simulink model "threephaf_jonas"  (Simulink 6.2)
settings: Solver=ode23  StartTime=0  StopTime=0.05  FixedStep=0.000001  MaxStep=2e-5  RelTol=1e-3
undefined symbols (not defined in the file or in its folder): Cdc, di, DiscIntNeverNeededParam, Element, L, R, Symmetrized, Tf, Ts, Udc, Upp, Warning, Yes
libraries: simulink x12
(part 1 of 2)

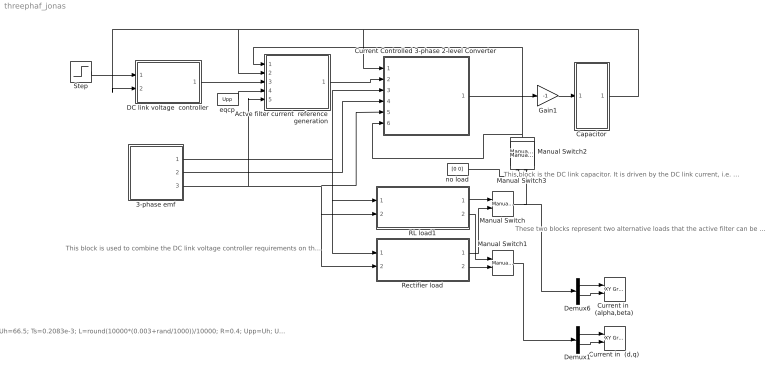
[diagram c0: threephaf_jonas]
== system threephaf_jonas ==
  note: These two blocks represent two alternative loads that the active filter can be used with.
  note: This block is the DC link capacitor. It is driven by the DC link current, i.e. the DC link voltage is the integral of the DC link current divided by the capacitance.
  note: This block is used to combine the DC link voltage controller requirements on the filter current with the components of the load current that can be filtered out.
  note: Uh=66.5; Ts=0.2083e-3; L=round(10000*(0.003+rand/1000))/10000; R=0.4; Upp=Uh; Udc=250; Cdc=0.0011; di=3; Tf=1/(2*pi*30);
  3-phase emf : Subsystem  mask{Upp=Upp, freq=50, Tc=0.1e-3}
      mask prompts: Upp "U_phase_to_phase [RMS]"; freq "Frequency"; Tc "Sampling time"
  Actve filter current  reference generation : Subsystem
  Capacitor : Subsystem
  Current Controlled 3-phase 2-level Converter : Subsystem
  Current in  (alpha,beta) : simulink/Sinks/XY Graph  xmin=-20  xmax=20  ymin=-20  ymax=20  st=-1
  Current in  (d,q) : simulink/Sinks/XY Graph  xmin=-20  xmax=20  ymin=-20  ymax=20  st=-1
  DC link voltage  controller : Subsystem  mask{Kp=Cdc/3/Tf, Ti=9*Tf, Ttc=Ts, Limitoutput=Yes, Out_max=20, Out_min=-20}
      mask prompts: Kp "Gain"; Ti "Integral time constant"; Ttc "Controller Sampling Time"; Limitoutput "Limit the output"; Out_max "Max Controller Output (if limited)     INCLUDES Anti Windup !!"; Out_min "Min Controller Output (if limited)     INCLUDES Anti Windup !!"
  Demux1 : Demux  Outputs=2
  Demux6 : Demux  Outputs=2
  Gain1 : Gain  Gain=-1
  Manual Switch : simulink/Signal Routing/Manual Switch  sw=1  action=0
  Manual Switch1 : simulink/Signal Routing/Manual Switch  sw=1  action=0
  Manual Switch2 : simulink/Signal Routing/Manual Switch  Orientation=up  sw=1  action=0
  Manual Switch3 : simulink/Signal Routing/Manual Switch  Orientation=up  sw=0  action=0
  RL load1 : Subsystem  mask{Ra=5, Rb=5, Rc=5, La=0.005, Lb=0.005, Lc=0.005, Imax=1}
      mask prompts: Ra "Ra [Ohm]"; Rb "Rb [Ohm]"; Rc "Rc [Ohm]"; La "La [H]"; Lb "Lb [H]"; Lc "Lc [H]"; Imax "Current when saturation starts"
  Rectifier load : Subsystem
  Step : Step  Time=0.005  Before=250  After=260  SampleTime=0
  eqcp : Constant  Value=Upp
  no load : Constant  Value=[0 0]
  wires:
  Gain1/1 -> Capacitor/1(iC)
  Current Controlled 3-phase 2-level Converter/1(idc) -> Gain1/1
  DC link voltage  controller/1(Out) -> Actve filter current  reference generation/3(idc*)
  eqcp/1 -> Actve filter current  reference generation/4(eqcp)
  Step/1 -> DC link voltage  controller/1(Ref)
  Capacitor/1(Udc) -> Actve filter current  reference generation/2(Udc), DC link voltage  controller/2(Act), Current Controlled 3-phase 2-level Converter/1(Udc)
  RL load1/1(i_load_ab) -> Manual Switch/1
  Rectifier load/1(i_load_ab) -> Manual Switch/2
  Rectifier load/2(i_load_dq) -> Manual Switch1/2
  RL load1/2(i_load_dq) -> Manual Switch1/1
  Actve filter current  reference generation/1(idq*) -> Current Controlled 3-phase 2-level Converter/2(idq*)
  3-phase emf/1(e_line) -> Current Controlled 3-phase 2-level Converter/3(e_line), Rectifier load/1(u_line), RL load1/1(u_line)
  3-phase emf/2(Psi_line) -> Current Controlled 3-phase 2-level Converter/4(Psi_line)
  3-phase emf/3(Theta_line) -> Actve filter current  reference generation/5(Theta), Current Controlled 3-phase 2-level Converter/5(Theta_line), Rectifier load/2(Theta), RL load1/2(Theta)
  Manual Switch/1 -> Manual Switch2/2, Demux6/1
  no load/1 -> Manual Switch2/1
  Manual Switch2/1 -> Actve filter current  reference generation/1(i_load), Current Controlled 3-phase 2-level Converter/6(Load current in a/b)
  Manual Switch1/1 -> Demux1/1
  Demux6/1 -> Current in  (alpha,beta)/1
  Demux6/2 -> Current in  (alpha,beta)/2
  Demux1/1 -> Current in  (d,q)/1
  Demux1/2 -> Current in  (d,q)/2

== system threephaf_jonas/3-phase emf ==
  note: Power invariant emf vector on alpha/beta frame
  Cos Fcn : Fcn  Expr=cos(2*pi*(u(2))*u(1))
  Digital Clock : DigitalClock  SampleTime=Tc
  Mux : Mux  Inputs=2
  Mux1 : Mux  Inputs=2
  Product : Product
  Sine Fcn : Fcn  Expr=sin(2*pi*(u(2))*u(1)-pi)
  frequency : Constant  Value=freq
  integrator : Subsystem
  line voltage : Constant  Value=Upp
  rec_to_pol : Subsystem
  e_line : Outport  InitialOutput=0
  Psi_line : Outport  Port=2  InitialOutput=0
  Theta_line : Outport  Port=3  InitialOutput=0
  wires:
  Product/1 -> e_line/1, integrator/1(In1)
  Mux1/1 -> Product/1
  Cos Fcn/1 -> Mux1/2
  Sine Fcn/1 -> Mux1/1
  Mux/1 -> Cos Fcn/1, Sine Fcn/1
  Digital Clock/1 -> Mux/1
  frequency/1 -> Mux/2
  line voltage/1 -> Product/2
  integrator/1(Out1) -> Psi_line/1, rec_to_pol/1(rect)
  rec_to_pol/2(angle) -> Theta_line/1

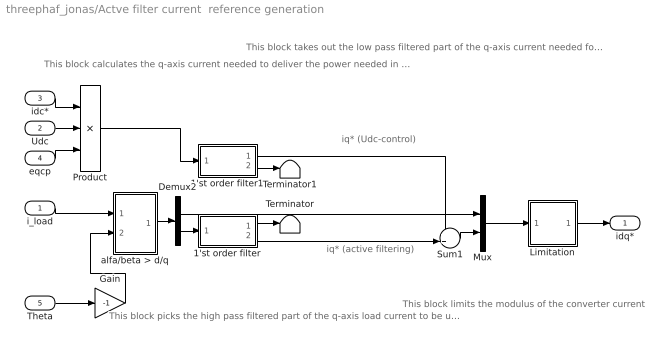
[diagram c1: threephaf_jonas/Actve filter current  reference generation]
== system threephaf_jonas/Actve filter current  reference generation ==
  note: iq* (Udc-control)
  note: iq* (active filtering)
  note: This block calculates the q-axis current needed to deliver the power needed in the dc-link for correcting the DC link voltage error, as ordered by the DC link voltage controller
  note: This block takes out the low pass filtered part of the q-axis current needed for DC link voltage control
  note: This block picks the high pass filtered part of the q-axis load current to be used as reference for the q-axis together with the low pass filtered part of the DC link voltage controller output.
  note: This block limits the modulus of the converter current
  i_load : Inport  Port=1  LatchInput=off
  Udc : Inport  Port=2  LatchInput=off
  idc* : Inport  Port=3  LatchInput=off
  eqcp : Inport  Port=4  LatchInput=off
  Theta : Inport  Port=5  LatchInput=off
  1'st order filter : Subsystem
  1'st order filter1 : Subsystem
  Demux2 : Demux  Outputs=2
  Gain : Gain  Gain=-1
  Limitation : Subsystem
  Mux : Mux  Inputs=2
  Product : Product  Inputs=**/
  Sum1 : Sum  Inputs=++|
  Terminator : Terminator
  Terminator1 : Terminator
  alfa/beta > d/q : Subsystem
  idq* : Outport
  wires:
  i_load/1 -> alfa/beta > d/q/1(vect)
  Gain/1 -> alfa/beta > d/q/2(angle)
  Theta/1 -> Gain/1
  Demux2/1 -> Mux/1
  Demux2/2 -> 1'st order filter/1(In)
  1'st order filter/1(OutLP) -> Terminator/1
  alfa/beta > d/q/1(Out) -> Demux2/1
  1'st order filter/2(OutHP) -> Sum1/2
  Sum1/1 -> Mux/2
  Limitation/1(i*lim) -> idq*/1
  1'st order filter1/1(OutLP) -> Sum1/1
  eqcp/1 -> Product/3
  Udc/1 -> Product/2
  Product/1 -> 1'st order filter1/1(In)
  idc*/1 -> Product/1
  1'st order filter1/2(OutHP) -> Terminator1/1
  Mux/1 -> Limitation/1(i*)

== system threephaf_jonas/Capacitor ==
  iC : Inport  Port=1  LatchInput=off
  Gain : Gain  Gain=1/Cdc
  Integrator : Integrator  InitialCondition=Udc
  Udc : Outport
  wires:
  Gain/1 -> Integrator/1
  iC/1 -> Gain/1
  Integrator/1 -> Udc/1

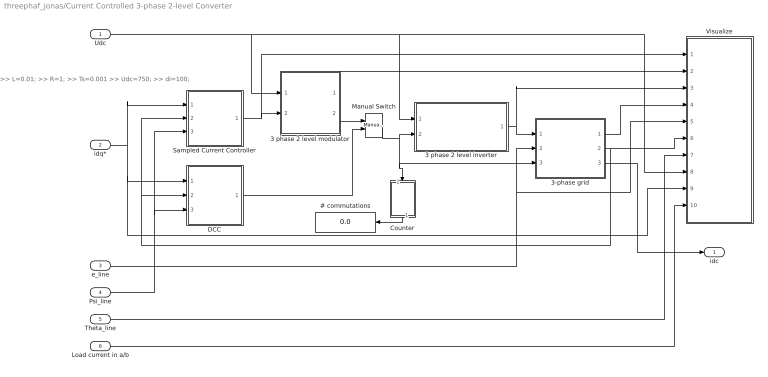
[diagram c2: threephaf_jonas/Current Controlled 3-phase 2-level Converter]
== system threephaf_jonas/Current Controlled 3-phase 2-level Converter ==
  note: >> L=0.01; >> R=1; >> Ts=0.001 >> Udc=750; >> di=100;
  Udc : Inport  Port=1  LatchInput=off
  idq* : Inport  Port=2  LatchInput=off
  e_line : Inport  Port=3  LatchInput=off
  Psi_line : Inport  Port=4  LatchInput=off
  Theta_line : Inport  Port=5  LatchInput=off
  Load current in a/b : Inport  Port=6  LatchInput=off
  # commutations : Display
  3 phase 2 level inverter : Subsystem
  3 phase 2 level modulator : Subsystem  mask{type=Symmetrized, Random=Fixed frequency, Ts=Ts}
      mask prompts: type "Sinus, Symmetrized or Minimum switch modulation"; Random "Fixed or random modulation?"; Ts "Sampling interval"
      mask help: Carrier Wave modulator that uses either fixed frequency modulation or random modulation. The fixed frequency modulation uses 1/(2Ts) as modulation frequency. The random modulation selects the modulatio frequency by random every sampling instant. The selection uses either 1/Ts, 1/(2Ts) or 1/(3Ts) as carrier wave frequency.
  3-phase grid : Subsystem  mask{L=L, R=R}
      mask prompts: L "Inductance [H]"; R "Resistance [ohm]"
  Counter : Subsystem  Orientation=down
  DCC : Subsystem
  Manual Switch : simulink/Signal Routing/Manual Switch  sw=1  action=0
  Sampled Current Controller : Subsystem  mask{R=R, L=L, Kp=(L/Ts+R/2), Ti=L/R+Ts/2, Ts=Ts, Umax=Udc, Umin=-Udc, SlowFast=Fast computer}
      mask prompts: R "Load resistance"; L "Load inductance"; Kp "Controller gain"; Ti "Integral Time Constant"; Ts "Sampling time [s]"; Umax "Max output signal"; Umin "Min output signal"; SlowFast "Controller type"
  Visualize : Subsystem
  idc : Outport
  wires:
  3 phase 2 level inverter/1(va,b,c) -> 3-phase grid/1(va,b,c), Visualize/3(v)
  Sampled Current Controller/1(u*) -> 3 phase 2 level modulator/2(uabc*), Visualize/1(u*)
  Udc/1 -> 3 phase 2 level modulator/1(Udc), 3 phase 2 level inverter/1(Udc), Visualize/8(Udc)
  Counter/1(#) -> # commutations/1
  3 phase 2 level modulator/2(sa,b,c) -> Manual Switch/1
  Manual Switch/1 -> 3 phase 2 level inverter/2(sa,b,c), Counter/1(sa,b,c), 3-phase grid/3(s)
  DCC/1(sa,b,c) -> Manual Switch/2
  3 phase 2 level modulator/1(mod) -> Visualize/2(mod)
  e_line/1 -> 3-phase grid/2(e_line), Visualize/5(e)
  3-phase grid/1(u_ab) -> Visualize/4("u ")
  3-phase grid/2(i_ab) -> Visualize/6(i), DCC/2(Act_ab), Sampled Current Controller/2(Act_ab)
  Theta_line/1 -> Visualize/7(theta)
  Psi_line/1 -> DCC/3(psi), Sampled Current Controller/3(psi)
  idq*/1 -> Sampled Current Controller/1(Ref_dq), DCC/1(Ref_dq), Visualize/9(i*dq)
  3-phase grid/3(i_dc) -> idc/1
  Load current in a/b/1 -> Visualize/10(Load current in a/b)

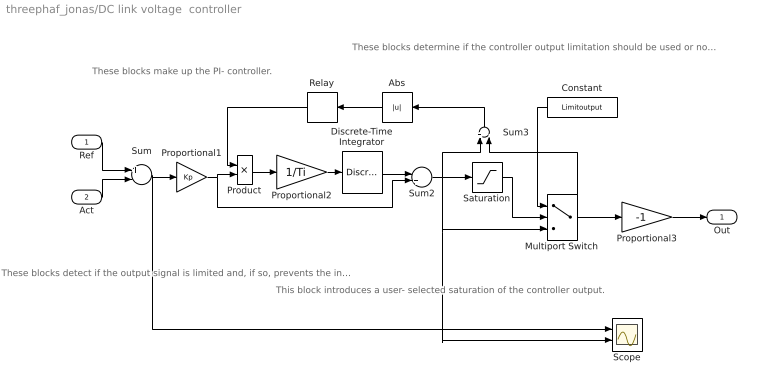
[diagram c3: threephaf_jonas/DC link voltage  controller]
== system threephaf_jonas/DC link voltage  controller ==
  note: These blocks make up the PI- controller.
  note: These blocks detect if the output signal is limited and, if so, prevents the integrator from integrating.
  note: This block introduces a user- selected saturation of the controller output.
  note: These blocks determine if the controller output limitation should be used or not.
  Ref : Inport  Port=1  LatchInput=off
  Act : Inport  Port=2  LatchInput=off
  Abs : Abs  Orientation=left
  Constant : Constant  Orientation=left  Value=Limitoutput
  Discrete-Time Integrator : DiscreteIntegrator  SampleTime=Ttc  ICPrevOutput=DiscIntNeverNeededParam  ICPrevScaledInput=DiscIntNeverNeededParam
  Multiport Switch : MultiPortSwitch  Inputs=2
  Product : Product
  Proportional1 : Gain  Gain=Kp
  Proportional2 : Gain  Gain=1/Ti
  Proportional3 : Gain  Gain=-1
  Relay : Relay  Orientation=left  OnOutputValue=0  OffOutputValue=1
  Saturation : Saturate  UpperLimit=Out_max  LowerLimit=Out_min
  Scope : Scope  NumInputPorts=2
  Sum : Sum  Inputs=+-
  Sum2 : Sum
  Sum3 : Sum  Orientation=up  Inputs=+-
  Out : Outport
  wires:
  Sum/1 -> Proportional1/1, Scope/1
  Discrete-Time Integrator/1 -> Sum2/1
  Proportional1/1 -> Product/2, Sum2/2
  Proportional2/1 -> Discrete-Time Integrator/1
  Sum2/1 -> Saturation/1, Sum3/1, Multiport Switch/3, Scope/2
  Product/1 -> Proportional2/1
  Sum3/1 -> Abs/1
  Abs/1 -> Relay/1
  Relay/1 -> Product/1
  Ref/1 -> Sum/1
  Act/1 -> Sum/2
  Saturation/1 -> Multiport Switch/2
  Constant/1 -> Multiport Switch/1
  Multiport Switch/1 -> Sum3/2, Proportional3/1
  Proportional3/1 -> Out/1

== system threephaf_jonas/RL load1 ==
  u_line : Inport  Port=1  LatchInput=off
  Theta : Inport  Port=2  LatchInput=off
  Gain1 : Gain  Gain=-1
  Load : Subsystem  mask{La=La, Lb=Lb, Lc=Lc, Imax=Imax, Ra=Ra, Rb=Rb, Rc=Rc}
      mask prompts: Imax "Inductor current for saturation"
  "a/b -> d/q1" : Subsystem
  abc Ü> vector : Subsystem
  vector to abc2 : Subsystem
  i_load_ab : Outport
  i_load_dq : Outport  Port=2
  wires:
  vector to abc2/1(a) -> Load/1(a)
  vector to abc2/2(b) -> Load/2(b)
  vector to abc2/3(c) -> Load/3(c)
  Load/1(ia) -> abc Ü> vector/1(a)
  Load/2(ib) -> abc Ü> vector/2(b)
  Load/3(ic) -> abc Ü> vector/3(c)
  u_line/1 -> vector to abc2/1(vect)
  abc Ü> vector/1(vect) -> i_load_ab/1, "a/b -> d/q1"/1(vect)
  Gain1/1 -> "a/b -> d/q1"/2(angle)
  Theta/1 -> Gain1/1
  "a/b -> d/q1"/1(Out) -> i_load_dq/1

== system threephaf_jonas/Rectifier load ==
  u_line : Inport  Port=1  LatchInput=off
  Theta : Inport  Port=2  LatchInput=off
  Gain1 : Gain  Gain=-1
  Load : Subsystem
  "a/b -> d/q1" : Subsystem
  abc Ü> vector : Subsystem
  vector to abc2 : Subsystem
  i_load_ab : Outport
  i_load_dq : Outport  Port=2
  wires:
  "a/b -> d/q1"/1(Out) -> i_load_dq/1
  Theta/1 -> Gain1/1
  Gain1/1 -> "a/b -> d/q1"/2(angle)
  vector to abc2/1(a) -> Load/1(a)
  vector to abc2/2(b) -> Load/2(b)
  vector to abc2/3(c) -> Load/3(c)
  Load/1(ia) -> abc Ü> vector/1(a)
  Load/2(ib) -> abc Ü> vector/2(b)
  Load/3(ic) -> abc Ü> vector/3(c)
  u_line/1 -> vector to abc2/1(vect)
  abc Ü> vector/1(vect) -> "a/b -> d/q1"/1(vect), i_load_ab/1

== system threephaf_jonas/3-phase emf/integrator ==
  note: Power invariant emf vector on alpha/beta frame
  In1 : Inport  Port=1  LatchInput=off
  Demux : Demux  Outputs=2
  Integrator1 : Integrator  InitialCondition=Upp/(2*pi*freq)
  Integrator2 : Integrator
  Mux : Mux  Inputs=2
  Out1 : Outport
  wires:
  In1/1 -> Demux/1
  Mux/1 -> Out1/1
  Integrator2/1 -> Mux/2
  Integrator1/1 -> Mux/1
  Demux/2 -> Integrator2/1
  Demux/1 -> Integrator1/1

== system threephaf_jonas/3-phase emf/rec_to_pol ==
  rect : Inport  Port=1  LatchInput=off
  Derivative : Derivative
  Gain : Gain  Gain=-1
  alfa/beta Ü> d/q : Subsystem
  "angle " : Fcn  Expr=atan2(u[2],u[1])
  "mod " : Fcn  Expr=sqrt(u[1]^2+u[2]^2)
  e : Outport  InitialOutput=0
  angle : Outport  Port=2  InitialOutput=0
  mod : Outport  Port=3  InitialOutput=0
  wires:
  "angle "/1 -> angle/1, Gain/1
  rect/1 -> "angle "/1, "mod "/1, Derivative/1
  "mod "/1 -> mod/1
  Gain/1 -> alfa/beta Ü> d/q/2(angle)
  Derivative/1 -> alfa/beta Ü> d/q/1(vect)
  alfa/beta Ü> d/q/1(Out) -> e/1

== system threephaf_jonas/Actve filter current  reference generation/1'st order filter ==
  In : Inport  Port=1  LatchInput=off
  Gain4 : Gain  Gain=1/Tf
  Integrator : Integrator
  Sum : Sum  Inputs=-+
  Sum4 : Sum  Inputs=+-
  OutLP : Outport
  OutHP : Outport  Port=2
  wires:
  Sum4/1 -> Gain4/1
  Gain4/1 -> Integrator/1
  Integrator/1 -> OutLP/1, Sum4/2, Sum/1
  In/1 -> Sum4/1, Sum/2
  Sum/1 -> OutHP/1

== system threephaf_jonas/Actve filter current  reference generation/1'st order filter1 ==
  In : Inport  Port=1  LatchInput=off
  Gain : Gain  Gain=1/(Tf)
  Integrator : Integrator
  Sum : Sum  Inputs=-+
  Sum1 : Sum  Inputs=|+-
  OutLP : Outport
  OutHP : Outport  Port=2
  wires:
  Sum1/1 -> Gain/1
  Gain/1 -> Integrator/1
  Integrator/1 -> OutLP/1, Sum1/2, Sum/1
  In/1 -> Sum1/1, Sum/2
  Sum/1 -> OutHP/1

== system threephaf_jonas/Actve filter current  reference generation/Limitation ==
  note: abs(i*)
  note: Current Limiter
  i* : Inport  Port=1  LatchInput=off
  Constant : Constant  Value=20*sqrt(3/2)
  Fcn1 : Fcn  Expr=sqrt(u(1)^2+u(2)^2)
  Product : Product
  Product1 : Product
  Saturation : Saturate  UpperLimit=1  LowerLimit=0
  Sign4 : Signum
  Sum2 : Sum  Inputs=-+
  Switch4 : Switch
  i*lim : Outport
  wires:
  Saturation/1 -> Product1/2
  Product/1 -> Saturation/1
  Switch4/1 -> Product/1
  Fcn1/1 -> Product/2, Switch4/3, Sum2/2
  Sum2/1 -> Sign4/1
  Sign4/1 -> Switch4/2
  Constant/1 -> Switch4/1, Sum2/1
  i*/1 -> Product1/1, Fcn1/1
  Product1/1 -> i*lim/1

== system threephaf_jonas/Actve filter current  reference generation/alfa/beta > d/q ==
  vect : Inport  Port=1  LatchInput=off
  angle : Inport  Port=2  LatchInput=off
  Fcn : Fcn  Expr=u[1]*cos(u[3])-u[2]*sin(u[3])
  Fcn1 : Fcn  Expr=u[1]*sin(u[3])+u[2]*cos(u[3])
  Mux : Mux  Inputs=2
  Mux1 : Mux  Inputs=2
  Out : Outport  InitialOutput=0
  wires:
  vect/1 -> Mux/1
  angle/1 -> Mux/2
  Mux/1 -> Fcn/1, Fcn1/1
  Fcn/1 -> Mux1/1
  Fcn1/1 -> Mux1/2
  Mux1/1 -> Out/1

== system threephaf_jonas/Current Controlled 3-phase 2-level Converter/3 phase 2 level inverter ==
  Udc : Inport  Port=1  LatchInput=off
  sa,b,c : Inport  Port=2  LatchInput=off
  Demux : Demux  Outputs=3
  Gain : Gain  Gain=1/2
  Gain1 : Gain  Gain=-1/2
  Mux : Mux  Orientation=down  Inputs=3
  Switch : Switch
  Switch1 : Switch
  Switch2 : Switch
  va,b,c : Outport  Orientation=down  InitialOutput=0
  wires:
  Gain/1 -> Switch/1, Switch1/1, Switch2/1
  Gain1/1 -> Switch/3, Switch1/3, Switch2/3
  Udc/1 -> Gain1/1, Gain/1
  sa,b,c/1 -> Demux/1
  Demux/1 -> Switch/2
  Demux/2 -> Switch1/2
  Demux/3 -> Switch2/2
  Switch/1 -> Mux/1
  Switch1/1 -> Mux/2
  Switch2/1 -> Mux/3
  Mux/1 -> va,b,c/1

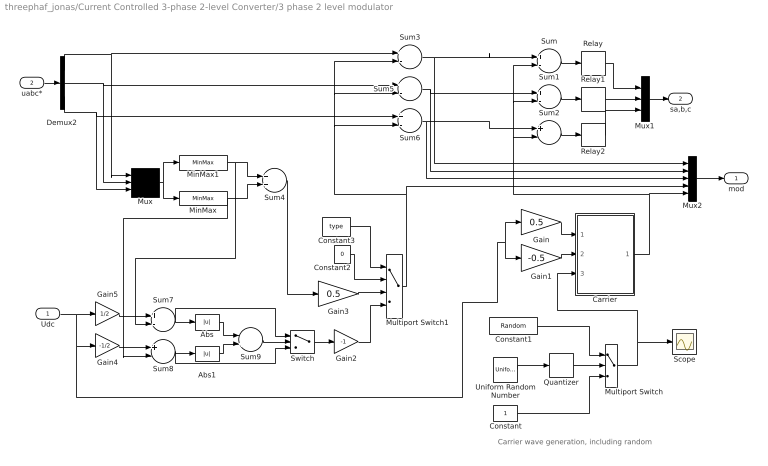
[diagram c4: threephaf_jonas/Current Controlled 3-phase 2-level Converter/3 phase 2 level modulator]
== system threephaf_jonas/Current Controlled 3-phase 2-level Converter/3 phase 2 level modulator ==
  note: Carrier wave generation, including random
  Udc : Inport  Port=1  LatchInput=off
  uabc* : Inport  Port=2  LatchInput=off
  Abs : Abs
  Abs1 : Abs
  Carrier : Subsystem
  Constant : Constant
  Constant1 : Constant  Value=Random
  Constant2 : Constant  Value=0
  Constant3 : Constant  Value=type
  Demux2 : Demux  Outputs=3
  Gain : Gain  Gain=0.5
  Gain1 : Gain  Gain=-0.5
  Gain2 : Gain  Gain=-1
  Gain3 : Gain  Gain=0.5
  Gain4 : Gain  Gain=-1/2
  Gain5 : Gain  Gain=1/2
  MinMax : MinMax
  MinMax1 : MinMax  Function=max
  Multiport Switch : MultiPortSwitch  Inputs=2
  Multiport Switch1 : MultiPortSwitch  Inputs=3
  Mux : Mux  Inputs=3
  Mux1 : Mux  Inputs=3
  Mux2 : Mux  Inputs=5
  Quantizer : Quantizer  QuantizationInterval=1
  Relay : Relay  OffOutputValue=-1
  Relay1 : Relay  OffOutputValue=-1
  Relay2 : Relay  OffOutputValue=-1
  Scope : Scope
  Sum{,1..3,5..8} (8 alike) : Sum  Inputs=+-
  Sum4 : Sum
  Sum9 : Sum  Inputs=-+
  Switch : Switch
  Uniform Random Number : UniformRandomNumber  Minimum=1  Maximum=3  Seed=0.9874  SampleTime=Ts
  mod : Outport  InitialOutput=0
  sa,b,c : Outport  Port=2  InitialOutput=0
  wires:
  Carrier/1(um) -> Sum2/2, Sum1/2, Sum/2, Mux2/5
  Gain1/1 -> Carrier/2(Umin)
  Gain/1 -> Carrier/1(Umax)
  Sum/1 -> Relay/1
  Relay1/1 -> Mux1/2
  Sum1/1 -> Relay1/1
  Relay2/1 -> Mux1/3
  Sum2/1 -> Relay2/1
  Sum3/1 -> Mux2/1, Sum/1
  Sum5/1 -> Mux2/2, Sum1/1
  Sum6/1 -> Mux2/3, Sum2/1
  Demux2/1 -> Sum3/1, Mux/1
  Demux2/2 -> Sum5/1, Mux/2
  Demux2/3 -> Sum6/1, Mux/3
  Mux/1 -> MinMax1/1, MinMax/1
  MinMax1/1 -> Sum4/1, Sum7/2
  MinMax/1 -> Sum4/2, Sum8/2
  Udc/1 -> Gain5/1, Gain4/1, Gain1/1, Gain/1
  Gain4/1 -> Sum8/1
  Sum7/1 -> Abs/1, Switch/1
  Sum8/1 -> Abs1/1, Switch/3
  Abs/1 -> Sum9/1
  Abs1/1 -> Sum9/2
  Sum9/1 -> Switch/2
  Sum4/1 -> Gain3/1
  Switch/1 -> Gain2/1
  Constant3/1 -> Multiport Switch1/1
  Constant2/1 -> Multiport Switch1/2
  Gain3/1 -> Multiport Switch1/3
  Gain2/1 -> Multiport Switch1/4
  Multiport Switch1/1 -> Sum5/2, Sum3/2, Sum6/2, Mux2/4
  Gain5/1 -> Sum7/1
  uabc*/1 -> Demux2/1
  Relay/1 -> Mux1/1
  Mux1/1 -> sa,b,c/1
  Mux2/1 -> mod/1
  Quantizer/1 -> Multiport Switch/2
  Uniform Random Number/1 -> Quantizer/1
  Constant/1 -> Multiport Switch/3
  Multiport Switch/1 -> Scope/1, Carrier/3(x)
  Constant1/1 -> Multiport Switch/1

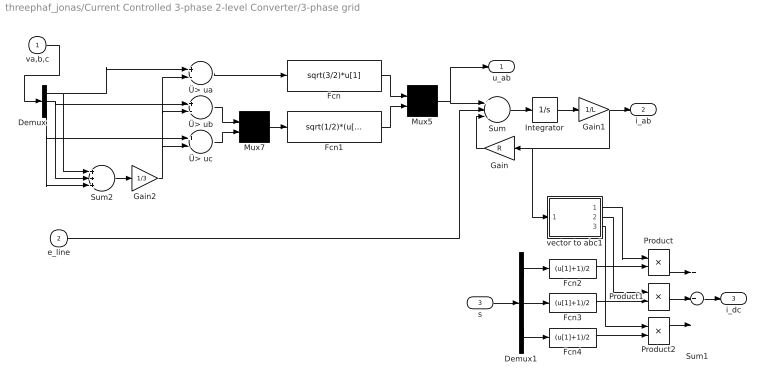
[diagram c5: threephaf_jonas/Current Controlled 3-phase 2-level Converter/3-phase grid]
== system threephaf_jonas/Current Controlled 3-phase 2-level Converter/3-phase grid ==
  va,b,c : Inport  Port=1  LatchInput=off
  e_line : Inport  Port=2  LatchInput=off
  s : Inport  Port=3  LatchInput=off
  Demux : Demux  Outputs=3
  Demux1 : Demux  Outputs=3
  Fcn : Fcn  Expr=sqrt(3/2)*u[1]
  Fcn1 : Fcn  Expr=sqrt(1/2)*(u[1]-u[2])
  Fcn2 : Fcn  Expr=(u[1]+1)/2
  Fcn3 : Fcn  Expr=(u[1]+1)/2
  Fcn4 : Fcn  Expr=(u[1]+1)/2
  Gain : Gain  Orientation=left  Gain=R
  Gain1 : Gain  Gain=1/L
  Gain2 : Gain  Gain=1/3
  Integrator : Integrator
  Mux5 : Mux  Inputs=2
  Mux7 : Mux  Inputs=2
  Product : Product
  Product1 : Product
  Product2 : Product
  Sum : Sum  Inputs=+--
  Sum1 : Sum  Inputs=+++
  Sum2 : Sum  Inputs=+++
  vector to abc1 : Subsystem
  Ü> ua : Sum  Inputs=+-
  Ü> ub : Sum  Inputs=+-
  Ü> uc : Sum  Inputs=+-
  u_ab : Outport  InitialOutput=0
  i_ab : Outport  Port=2  InitialOutput=0
  i_dc : Outport  Port=3
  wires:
  Gain1/1 -> i_ab/1, Gain/1, vector to abc1/1(vect)
  Integrator/1 -> Gain1/1
  Gain/1 -> Sum/3
  Sum/1 -> Integrator/1
  Fcn1/1 -> Mux5/2
  Fcn/1 -> Mux5/1
  Mux5/1 -> Sum/1, u_ab/1
  Mux7/1 -> Fcn1/1
  Ü> uc/1 -> Mux7/2
  Ü> ub/1 -> Mux7/1
  Ü> ua/1 -> Fcn/1
  Gain2/1 -> Ü> uc/2, Ü> ub/2, Ü> ua/2
  Demux/2 -> Ü> ub/1, Sum2/2
  Sum2/1 -> Gain2/1
  Demux/3 -> Ü> uc/1, Sum2/3
  Demux/1 -> Ü> ua/1, Sum2/1
  va,b,c/1 -> Demux/1
  Demux1/2 -> Fcn3/1
  Demux1/1 -> Fcn2/1
  Demux1/3 -> Fcn4/1
  s/1 -> Demux1/1
  Sum1/1 -> i_dc/1
  Product2/1 -> Sum1/3
  Product1/1 -> Sum1/2
  Product/1 -> Sum1/1
  vector to abc1/1(a) -> Product/1
  vector to abc1/2(b) -> Product1/1
  vector to abc1/3(c) -> Product2/1
  Fcn4/1 -> Product2/2
  Fcn3/1 -> Product1/2
  Fcn2/1 -> Product/2
  e_line/1 -> Sum/2

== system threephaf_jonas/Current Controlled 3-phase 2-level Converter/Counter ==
  sa,b,c : Inport  Port=1  LatchInput=off
  Demux : Demux  Outputs=3
  Subsystem : Subsystem  TreatAsAtomicUnit=on
  Subsystem1 : Subsystem  TreatAsAtomicUnit=on
  Subsystem2 : Subsystem  TreatAsAtomicUnit=on
  Sum : Sum  Inputs=+++
  # : Outport
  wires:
  Sum/1 -> #/1
  Subsystem/1(Out1) -> Sum/2
  Subsystem2/1(Out1) -> Sum/1
  Subsystem1/1(Out1) -> Sum/3
  sa,b,c/1 -> Demux/1
  Demux/2 -> Subsystem/Trigger
  Demux/3 -> Subsystem1/Trigger
  Demux/1 -> Subsystem2/Trigger

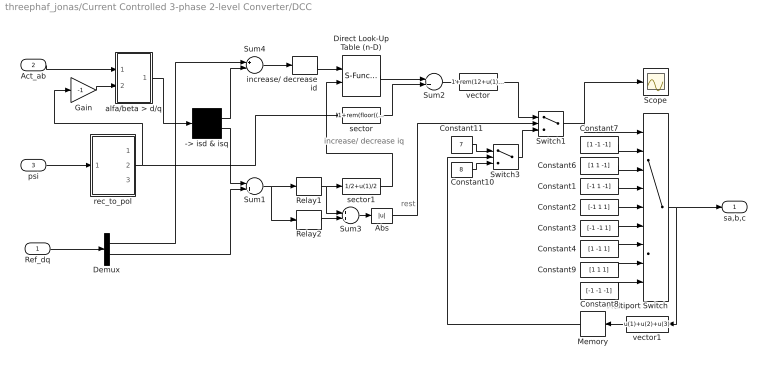
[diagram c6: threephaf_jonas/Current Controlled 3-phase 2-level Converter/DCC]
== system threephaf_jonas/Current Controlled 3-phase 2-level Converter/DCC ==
  note: increase/ decrease iq
  note: rest
  Ref_dq : Inport  Port=1  LatchInput=off
  Act_ab : Inport  Port=2  LatchInput=off
  psi : Inport  Port=3  LatchInput=off
  -> isd & isq : Demux  Outputs=2
  Abs : Abs
  Constant1 : Constant  Value=[-1 1 -1]
  Constant10 : Constant  Value=8
  Constant11 : Constant  Value=7
  Constant2 : Constant  Value=[-1 1 1]
  Constant3 : Constant  Value=[-1 -1 1]
  Constant4 : Constant  Value=[1 -1 1]
  Constant6 : Constant  Value=[1 1 -1]
  Constant7 : Constant  Value=[1 -1 -1]
  Constant8 : Constant  Value=[-1 -1 -1]
  Constant9 : Constant  Value=[1 1 1]
  Demux : Demux  Outputs=2
  Direct Look-Up Table (n-D) : S-Function  FunctionName=sfun_nddirectlook  Parameters=numInputs,mxTable,clipFlag,tabIsInput,numTDims  mask(LookupNDDirect){maskTabDims=2, explicitNumDims=1, outDims=Element, tabIsInput=off, mxTable=[4 2;5 1], clipFlag=Warning}
      mask prompts: maskTabDims "Number of table dimensions:"; explicitNumDims "Explicit number of table dimensions:"; outDims "Inputs select this object from table:"; tabIsInput "Make table an input"; mxTable "Table data:"; clipFlag "Action for out of range input:"
      mask help: Table member selection. Inputs are zero-based indices into the table, e.g., an input of 3 returns the fourth element in that dimension. Block can also be used to select a column or 2-D matrix out of the table.
      mask init:
      | if tabIsInput == 1
      |   tWhat = ' T';
      |   yT = 1/(3+maskTabDims-outDims);
      | else
      |   tWhat = ' ';
      |   yT = 0;
      | end
      | if maskTabDims >= 5
      |   numTDims = explicitNumDims;
      | else
      |   numTDims = maskTabDims;
      | end
      | numInputs =  numTDims - (outDims-1);
      | if strcmp(get_param(bdroot(gcb),'BlockDiagramType'),'library')
      |   dimsChar = 'n';
      | else
      |   dimsChar = sprintf('%d',numTDims);
      | end
      | [x,y] = nddirectico('plotdata', numTDims, tabIsInput, outDims);
      | xp = x((end-3):end); yp = y((end-3):end);
      | x = x(1:(end-4)); y = y(1:(end-4));
  Gain : Gain  Gain=-1
  Memory : Memory  Orientation=left
  Multiport Switch : MultiPortSwitch  Inputs=8
  Relay1 : Relay  OnSwitchValue=di/2  OffSwitchValue=-di/2  OffOutputValue=-1
  Relay2 : Relay  OnSwitchValue=1.3*di/2  OffSwitchValue=-1.3*di/2  OffOutputValue=-1
  Scope : Scope
  Sum1 : Sum  Inputs=-+
  Sum2 : Sum
  Sum3 : Sum
  Sum4 : Sum  Inputs=+-
  Switch1 : Switch  Threshold=1
  Switch3 : Switch  Threshold=1
  alfa/beta > d/q : Subsystem
  increase/ decrease id : Relay  OnSwitchValue=di/2  OffSwitchValue=-di/2
  rec_to_pol : Subsystem
  sector : Fcn  Expr=1+rem(floor((2*pi+u(1)+pi/6)/(pi/3+eps)),6)
  sector1 : Fcn  Expr=1/2+u(1)/2
  vector : Fcn  Expr=1+rem(12+u(1)-1,6)
  vector1 : Fcn  Orientation=left  Expr=u(1)+u(2)+u(3)
  sa,b,c : Outport
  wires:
  Gain/1 -> alfa/beta > d/q/2(angle)
  Act_ab/1 -> alfa/beta > d/q/1(vect)
  alfa/beta > d/q/1(Out) -> -> isd & isq/1
  psi/1 -> rec_to_pol/1(rect)
  -> isd & isq/1 -> Sum4/2
  rec_to_pol/2(angle) -> Gain/1, sector/1
  Multiport Switch/1 -> vector1/1, sa,b,c/1
  Switch1/1 -> Multiport Switch/1, Scope/1
  vector/1 -> Switch1/1
  Sum4/1 -> increase/ decrease id/1
  Sum2/1 -> vector/1
  vector1/1 -> Memory/1
  -> isd & isq/2 -> Sum1/1
  Constant10/1 -> Switch3/3
  Constant11/1 -> Switch3/1
  Memory/1 -> Switch3/2
  Switch3/1 -> Switch1/3
  Relay1/1 -> Sum3/1, sector1/1
  Relay2/1 -> Sum3/2
  Sum3/1 -> Abs/1
  Sum1/1 -> Relay1/1, Relay2/1
  Abs/1 -> Switch1/2
  increase/ decrease id/1 -> Direct Look-Up Table (n-D)/1
  sector1/1 -> Direct Look-Up Table (n-D)/2
  sector/1 -> Sum2/2
  Direct Look-Up Table (n-D)/1 -> Sum2/1
  Constant6/1 -> Multiport Switch/3
  Constant7/1 -> Multiport Switch/2
  Constant8/1 -> Multiport Switch/9
  Constant9/1 -> Multiport Switch/8
  Constant1/1 -> Multiport Switch/4
  Constant2/1 -> Multiport Switch/5
  Constant3/1 -> Multiport Switch/6
  Constant4/1 -> Multiport Switch/7
  Ref_dq/1 -> Demux/1
  Demux/1 -> Sum4/1
  Demux/2 -> Sum1/2

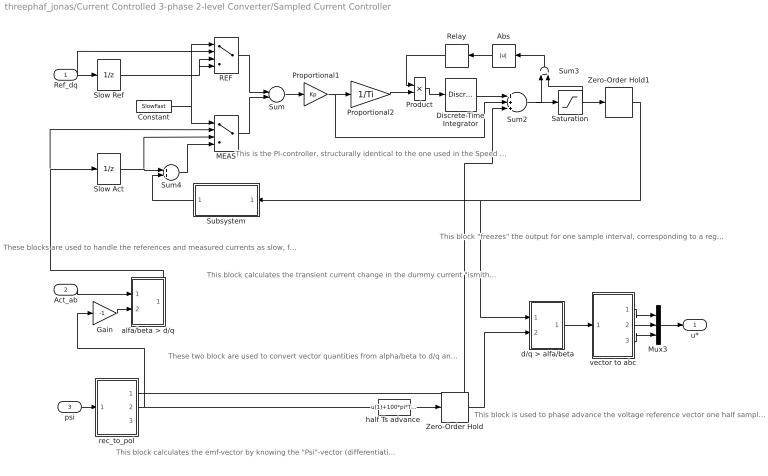
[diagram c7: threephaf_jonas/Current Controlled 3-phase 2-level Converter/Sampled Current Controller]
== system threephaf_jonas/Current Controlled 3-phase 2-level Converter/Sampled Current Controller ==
  note: These blocks are used to handle the references and measured currents as slow, fast or fast computer with Smith predictor.
  note: This block calculates the transient current change in the dummy current "ismith" The smith predictor calculates the current change that would have been measured if the computer was "fast", i.e. without the delay that a slow computer has. The calculated current change equals the real current change, but informing the controller one sampling interval earlier, thus allowing a high (deadbeat) gain.
  note: This is the PI-controller, structurally identical to the one used in the Speed Controller
  note: This block "freezes" the output for one sample interval, corresponding to a register in a microcontroller where the reference voltages are written once every sampling inteval.
  note: These two block are used to convert vector quantities from alpha/beta to d/q and back again. Note that they are identical, but use the angle with opposite sign.
  note: This block calculates the emf-vector by knowing the "Psi"-vector (differentiation) and calculates the emf- components in the d/q-plane (ideally there is only "eq" whilse "ed"=0). It alse calculates the angle of the "Psi"- vector, used to orient the d/q-plane.
  note: This block is used to phase advance the voltage reference vector one half sample period. It is done to compensate for the fact that the "reality" is turning during the same sample period as the voltage references are being held constant. In the beginning of the sample period, the voltage reference will be 1/2 sample period ahead of reality, and in the end of the sample period it will be 1/2 period behind. In average, it will be in the correct position relative to reality.
  Ref_dq : Inport  Port=1  LatchInput=off
  Act_ab : Inport  Port=2  LatchInput=off
  psi : Inport  Port=3  LatchInput=off
  " d/q > alfa/beta" : Subsystem
  Abs : Abs  Orientation=left
  Constant : Constant  Value=SlowFast
  Discrete-Time Integrator : DiscreteIntegrator  SampleTime=Ts  LimitOutput=on  UpperSaturationLimit=Umax  LowerSaturationLimit=Umin  ICPrevOutput=DiscIntNeverNeededParam  ICPrevScaledInput=DiscIntNeverNeededParam
  Gain : Gain  Gain=-1
  MEAS : MultiPortSwitch  Inputs=3
  Mux3 : Mux  Inputs=3
  Product : Product
  Proportional1 : Gain  Gain=Kp
  Proportional2 : Gain  Gain=1/Ti
  REF : MultiPortSwitch  Inputs=3
  Relay : Relay  Orientation=left  OnOutputValue=0  OffOutputValue=1
  Saturation : Saturate  UpperLimit=Umax  LowerLimit=Umin
  Slow Act : UnitDelay  SampleTime=Ts
  Slow Ref : UnitDelay  SampleTime=Ts
  Subsystem : Subsystem  Orientation=left
  Sum : Sum  Inputs=+-
  Sum2 : Sum  Inputs=+++
  Sum3 : Sum  Orientation=up  Inputs=+-
  Sum4 : Sum
  Zero-Order Hold : ZeroOrderHold  SampleTime=Ts
  Zero-Order Hold1 : ZeroOrderHold  SampleTime=Ts
  alfa/beta > d/q : Subsystem
  "half Ts advance " : Fcn  Expr=u(1)+100*pi*Ts/2
  rec_to_pol : Subsystem
  vector to abc : Subsystem
  u* : Outport
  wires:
  Discrete-Time Integrator/1 -> Sum2/1
  Proportional1/1 -> Proportional2/1, Sum2/2
  Sum/1 -> Proportional1/1
  Sum2/1 -> Saturation/1, Sum3/1
  Saturation/1 -> Zero-Order Hold1/1, Sum3/2
  Proportional2/1 -> Product/2
  Product/1 -> Discrete-Time Integrator/1
  Relay/1 -> Product/1
  Ref_dq/1 -> REF/2, Slow Ref/1
  Zero-Order Hold1/1 -> Subsystem/1(u), " d/q > alfa/beta"/1(vect)
  Slow Act/1 -> Sum4/1, MEAS/3
  Subsystem/1(di_smith) -> Sum4/2
  Constant/1 -> MEAS/1, REF/1
  Slow Ref/1 -> REF/3, REF/4
  REF/1 -> Sum/1
  Sum4/1 -> MEAS/4
  MEAS/1 -> Sum/2
  Sum3/1 -> Abs/1
  Abs/1 -> Relay/1
  Gain/1 -> alfa/beta > d/q/2(angle)
  Act_ab/1 -> alfa/beta > d/q/1(vect)
  psi/1 -> rec_to_pol/1(rect)
  rec_to_pol/2(angle) -> Gain/1, "half Ts advance "/1
  "half Ts advance "/1 -> Zero-Order Hold/1
  Zero-Order Hold/1 -> " d/q > alfa/beta"/2(angle)
  " d/q > alfa/beta"/1(Out) -> vector to abc/1(vect)
  vector to abc/1(a) -> Mux3/1
  vector to abc/2(b) -> Mux3/2
  vector to abc/3(c) -> Mux3/3
  alfa/beta > d/q/1(Out) -> Slow Act/1, MEAS/2
  Mux3/1 -> u*/1
  rec_to_pol/1(e) -> Sum2/3

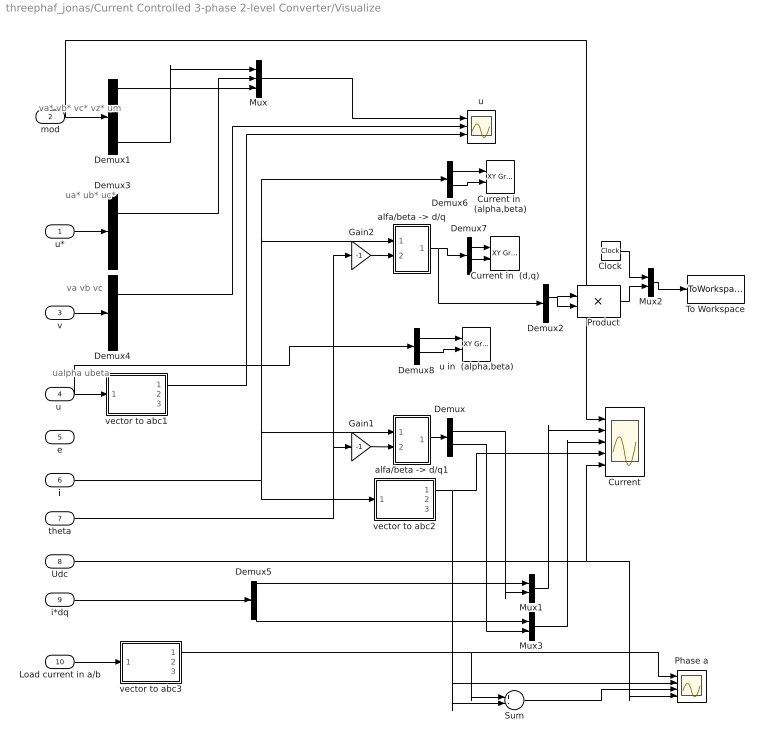
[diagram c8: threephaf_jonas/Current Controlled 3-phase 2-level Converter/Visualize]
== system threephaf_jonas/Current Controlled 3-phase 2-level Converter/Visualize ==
  note: va* vb* vc* vz* um
  note: ua* ub* uc*
  note: ualpha ubeta
  note: va vb vc
  u* : Inport  Port=1  LatchInput=off
  mod : Inport  Port=2  LatchInput=off
  v : Inport  Port=3  LatchInput=off
  "u " : Inport  Port=4  LatchInput=off
  e : Inport  Port=5  LatchInput=off
  i : Inport  Port=6  LatchInput=off
  theta : Inport  Port=7  LatchInput=off
  Udc : Inport  Port=8  LatchInput=off
  i*dq : Inport  Port=9  LatchInput=off
  Load current in a/b : Inport  Port=10  LatchInput=off
  Clock : Clock
  Current : Scope  NumInputPorts=5
  Current in  (alpha,beta) : simulink/Sinks/XY Graph  xmin=-20  xmax=20  ymin=-20  ymax=20  st=-1
  Current in  (d,q) : simulink/Sinks/XY Graph  xmin=-20  xmax=20  ymin=-20  ymax=20  st=-1
  Demux{,2,5..8} (6 alike) : Demux  Outputs=2
  Demux1 : Demux  Outputs=5
  Demux3 : Demux  Outputs=3
  Demux4 : Demux  Outputs=3
  Gain1 : Gain  Gain=-1
  Gain2 : Gain  Gain=-1
  Mux : Mux  Inputs=3
  Mux1 : Mux  Inputs=2
  Mux2 : Mux  Inputs=2
  Mux3 : Mux  Inputs=2
  Phase a : Scope  NumInputPorts=4
  Product : Product
  Sum : Sum  Inputs=+-
  To Workspace : ToWorkspace  VariableName=f1  SampleTime=-1  SaveFormat=Array
  "alfa/beta -> d/q" : Subsystem
  "alfa/beta -> d/q1" : Subsystem
  u : Scope  NumInputPorts=3
  u in  (alpha,beta) : simulink/Sinks/XY Graph  xmin=-300  xmax=300  ymin=-300  ymax=300  st=-1
  vector to abc1 : Subsystem
  vector to abc2 : Subsystem
  vector to abc3 : Subsystem
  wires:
  Gain2/1 -> "alfa/beta -> d/q"/2(angle)
  Gain1/1 -> "alfa/beta -> d/q1"/2(angle)
  "alfa/beta -> d/q1"/1(Out) -> Demux/1
  vector to abc2/1(a) -> Current/4, Phase a/2, Sum/2
  mod/1 -> Demux1/1, Current/1
  "alfa/beta -> d/q"/1(Out) -> Demux2/1, Demux7/1
  Demux1/5 -> Mux/1
  Demux1/1 -> Mux/3
  Mux/1 -> u/1
  u*/1 -> Demux3/1
  "u "/1 -> vector to abc1/1(vect), Demux8/1
  Demux3/1 -> Mux/2
  v/1 -> Demux4/1
  Demux4/1 -> u/2
  vector to abc1/1(a) -> u/3
  i/1 -> "alfa/beta -> d/q"/1(vect), Demux6/1, "alfa/beta -> d/q1"/1(vect), vector to abc2/1(vect)
  e/1 -> ?
  theta/1 -> Gain1/1, Gain2/1
  Clock/1 -> Mux2/1
  Product/1 -> Mux2/2
  Mux2/1 -> To Workspace/1
  Demux2/1 -> Product/1, Product/2
  Udc/1 -> Current/5, Phase a/4
  i*dq/1 -> Demux5/1
  Demux5/1 -> Mux1/1
  Demux5/2 -> Mux3/1
  Demux/1 -> Mux1/2
  Demux/2 -> Mux3/2
  Mux1/1 -> Current/2
  Mux3/1 -> Current/3
  Load current in a/b/1 -> vector to abc3/1(vect)
  vector to abc3/1(a) -> Phase a/1, Sum/1
  Sum/1 -> Phase a/3
  Demux6/1 -> Current in  (alpha,beta)/1
  Demux6/2 -> Current in  (alpha,beta)/2
  Demux7/1 -> Current in  (d,q)/1
  Demux7/2 -> Current in  (d,q)/2
  Demux8/1 -> u in  (alpha,beta)/1
  Demux8/2 -> u in  (alpha,beta)/2

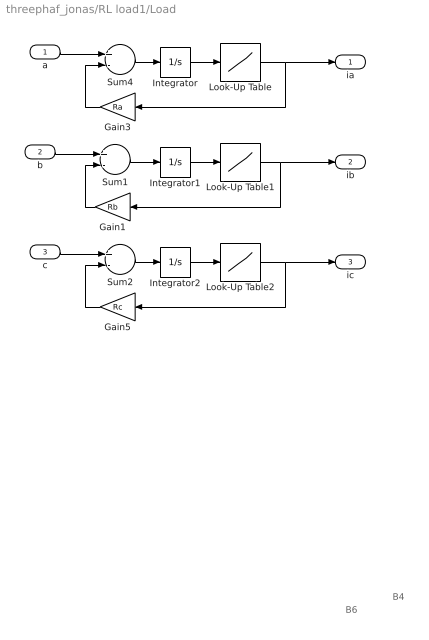
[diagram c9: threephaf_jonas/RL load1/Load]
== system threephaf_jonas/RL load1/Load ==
  note: B4
  note: B6
  a : Inport  Port=1  LatchInput=off
  b : Inport  Port=2  LatchInput=off
  c : Inport  Port=3  LatchInput=off
  Gain1 : Gain  Orientation=left  Gain=Rb
  Gain3 : Gain  Orientation=left  Gain=Ra
  Gain5 : Gain  Orientation=left  Gain=Rc
  Integrator : Integrator
  Integrator1 : Integrator
  Integrator2 : Integrator
  Look-Up Table : Lookup  InputValues=La*Imax*[-2 -1.5 -1 0 1 1.5 2]  OutputValues=Imax*[-10 -2 -1 0 1 2 10]
  Look-Up Table1 : Lookup  InputValues=Lb*Imax*[-2 -1.5 -1 0 1 1.5 2]  OutputValues=Imax*[-10 -2 -1 0 1 2 10]
  Look-Up Table2 : Lookup  InputValues=Lc*Imax*[-2 -1.5 -1 0 1 1.5 2]  OutputValues=Imax*[-10 -2 -1 0 1 2 10]
  Sum1 : Sum  Inputs=+-
  Sum2 : Sum  Inputs=+-
  Sum4 : Sum  Inputs=+-
  ia : Outport  InitialOutput=0
  ib : Outport  Port=2  InitialOutput=0
  ic : Outport  Port=3  InitialOutput=0
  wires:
  Gain3/1 -> Sum4/2
  Sum4/1 -> Integrator/1
  Integrator/1 -> Look-Up Table/1
  a/1 -> Sum4/1
  Gain1/1 -> Sum1/2
  Sum1/1 -> Integrator1/1
  Integrator1/1 -> Look-Up Table1/1
  b/1 -> Sum1/1
  Gain5/1 -> Sum2/2
  Sum2/1 -> Integrator2/1
  Integrator2/1 -> Look-Up Table2/1
  c/1 -> Sum2/1
  Look-Up Table/1 -> Gain3/1, ia/1
  Look-Up Table1/1 -> Gain1/1, ib/1
  Look-Up Table2/1 -> Gain5/1, ic/1

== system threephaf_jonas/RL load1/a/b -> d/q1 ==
  vect : Inport  Port=1  LatchInput=off
  angle : Inport  Port=2  LatchInput=off
  Fcn_x : Fcn  Expr=u[1]*cos(u[3])-u[2]*sin(u[3])
  Fcn_y : Fcn  Expr=u[1]*sin(u[3])+u[2]*cos(u[3])
  Mux : Mux  Inputs=2
  Mux1 : Mux  Inputs=2
  Out : Outport  InitialOutput=0
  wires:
  vect/1 -> Mux/1
  angle/1 -> Mux/2
  Mux/1 -> Fcn_x/1, Fcn_y/1
  Fcn_x/1 -> Mux1/1
  Fcn_y/1 -> Mux1/2
  Mux1/1 -> Out/1

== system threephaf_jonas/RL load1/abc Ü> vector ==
  a : Inport  Port=1  LatchInput=off
  b : Inport  Port=2  LatchInput=off
  c : Inport  Port=3  LatchInput=off
  Fcn : Fcn  Expr=sqrt(3/2)*u[1]
  Fcn1 : Fcn  Expr=sqrt(1/2)*(u[1]-u[2])
  Gain : Gain  Gain=1/3
  Mux5 : Mux  Inputs=2
  Mux7 : Mux  Inputs=2
  Sum2 : Sum  Inputs=+++
  Ü> ua : Sum  Inputs=+-
  Ü> ub : Sum  Inputs=+-
  Ü> uc : Sum  Inputs=+-
  vect : Outport  InitialOutput=0
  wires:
  Fcn1/1 -> Mux5/2
  Fcn/1 -> Mux5/1
  Mux5/1 -> vect/1
  Mux7/1 -> Fcn1/1
  Ü> uc/1 -> Mux7/2
  Ü> ub/1 -> Mux7/1
  Ü> ua/1 -> Fcn/1
  Gain/1 -> Ü> uc/2, Ü> ub/2, Ü> ua/2
  a/1 -> Ü> ua/1, Sum2/1
  b/1 -> Ü> ub/1, Sum2/2
  Sum2/1 -> Gain/1
  c/1 -> Ü> uc/1, Sum2/3

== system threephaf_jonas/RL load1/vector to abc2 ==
  vect : Inport  Port=1  LatchInput=off
  Ü> a : Fcn  Expr=sqrt(2/3)*u[1]
  Ü> b : Fcn  Expr=-sqrt(1/6)*u[1]+sqrt(1/2)*u[2]
  Ü> c : Fcn  Expr=-sqrt(1/6)*u[1]-sqrt(1/2)*u[2]
  a : Outport  InitialOutput=0
  b : Outport  Port=2  InitialOutput=0
  c : Outport  Port=3  InitialOutput=0
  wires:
  vect/1 -> Ü> b/1, Ü> a/1, Ü> c/1
  Ü> b/1 -> b/1
  Ü> c/1 -> c/1
  Ü> a/1 -> a/1

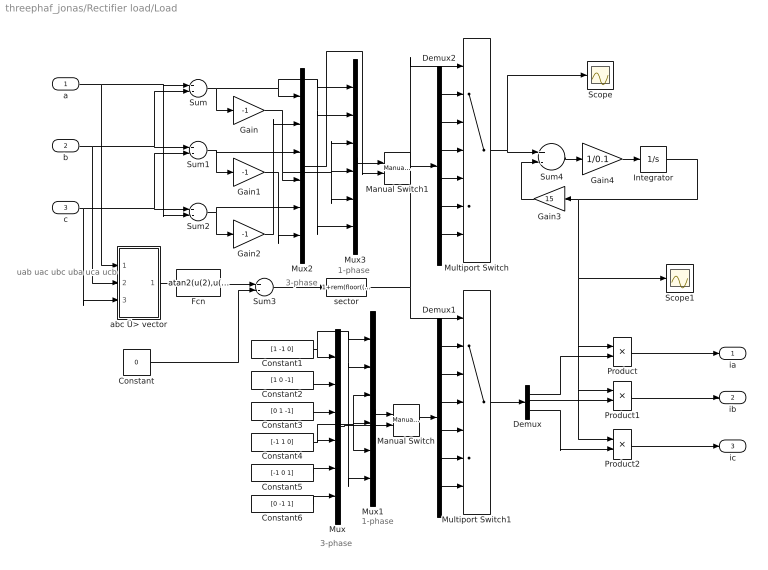
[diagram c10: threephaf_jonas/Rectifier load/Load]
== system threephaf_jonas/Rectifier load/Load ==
  note: uab uac ubc uba uca ucb
  note: 1-phase
  note: 3-phase
  note: 3-phase
  note: 1-phase
  a : Inport  Port=1  LatchInput=off
  b : Inport  Port=2  LatchInput=off
  c : Inport  Port=3  LatchInput=off
  Constant : Constant  Value=0
  Constant1 : Constant  Value=[1 -1 0]
  Constant2 : Constant  Value=[1 0 -1]
  Constant3 : Constant  Value=[0 1 -1]
  Constant4 : Constant  Value=[-1 1 0]
  Constant5 : Constant  Value=[-1 0 1]
  Constant6 : Constant  Value=[0 -1 1]
  Demux : Demux  Outputs=3
  Demux1 : Demux  Outputs=6
  Demux2 : Demux  Outputs=6
  Fcn : Fcn  Expr=atan2(u(2),u(1))
  Gain : Gain  Gain=-1
  Gain1 : Gain  Gain=-1
  Gain2 : Gain  Gain=-1
  Gain3 : Gain  Orientation=left  Gain=15
  Gain4 : Gain  Gain=1/0.1
  Integrator : Integrator  InitialCondition=400*sqrt(2)*3/pi/50
  Manual Switch : simulink/Signal Routing/Manual Switch  sw=0  action=0
  Manual Switch1 : simulink/Signal Routing/Manual Switch  sw=0  action=0
  Multiport Switch : MultiPortSwitch  Inputs=6
  Multiport Switch1 : MultiPortSwitch  Inputs=6
  Mux{,1..3} (4 alike) : Mux  Inputs=6
  Product : Product
  Product1 : Product
  Product2 : Product
  Scope : Scope
  Scope1 : Scope
  Sum{,1..4} (5 alike) : Sum  Inputs=+-
  abc Ü> vector : Subsystem
  sector : Fcn  Expr=1+rem(floor((2*pi+u(1)+pi/3)/(pi/3+eps)),6)
  ia : Outport  InitialOutput=0
  ib : Outport  Port=2  InitialOutput=0
  ic : Outport  Port=3  InitialOutput=0
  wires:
  Demux/3 -> Product2/2
  Demux/1 -> Product/2
  a/1 -> Sum/1, Sum2/2, abc Ü> vector/1(a)
  b/1 -> Sum1/1, Sum/2, abc Ü> vector/2(b)
  c/1 -> Sum2/1, Sum1/2, abc Ü> vector/3(c)
  Sum/1 -> Mux2/1, Mux3/2, Mux3/6, Mux3/1, Gain/1
  Sum1/1 -> Gain1/1, Mux2/3
  Sum2/1 -> Gain2/1, Mux2/5
  abc Ü> vector/1(vect) -> Fcn/1
  sector/1 -> Multiport Switch/1, Multiport Switch1/1
  Fcn/1 -> Sum3/1
  Sum3/1 -> sector/1
  Constant/1 -> Sum3/2
  Multiport Switch/1 -> Sum4/1, Scope/1
  Gain4/1 -> Integrator/1
  Gain3/1 -> Sum4/2
  Multiport Switch1/1 -> Demux/1
  Demux/2 -> Product1/2
  Product/1 -> ia/1
  Product1/1 -> ib/1
  Product2/1 -> ic/1
  Sum4/1 -> Gain4/1
  Integrator/1 -> Gain3/1, Product/1, Product1/1, Product2/1, Scope1/1
  Demux1/1 -> Multiport Switch1/2
  Demux1/2 -> Multiport Switch1/3
  Demux1/3 -> Multiport Switch1/4
  Demux1/4 -> Multiport Switch1/5
  Demux1/5 -> Multiport Switch1/6
  Demux1/6 -> Multiport Switch1/7
  Constant1/1 -> Mux/1, Mux1/2, Mux1/6, Mux1/1
  Constant2/1 -> Mux/2
  Constant3/1 -> Mux/3
  Constant4/1 -> Mux1/3, Mux1/4, Mux1/5, Mux/4
  Constant5/1 -> Mux/5
  Constant6/1 -> Mux/6
  Mux/1 -> Manual Switch/2
  Manual Switch/1 -> Demux1/1
  Mux1/1 -> Manual Switch/1
  Gain/1 -> Mux2/4, Mux3/3, Mux3/5, Mux3/4
  Gain1/1 -> Mux2/6
  Gain2/1 -> Mux2/2
  Demux2/1 -> Multiport Switch/2
  Demux2/2 -> Multiport Switch/3
  Demux2/3 -> Multiport Switch/4
  Demux2/4 -> Multiport Switch/5
  Demux2/5 -> Multiport Switch/6
  Demux2/6 -> Multiport Switch/7
  Mux3/1 -> Manual Switch1/1
  Manual Switch1/1 -> Demux2/1
  Mux2/1 -> Manual Switch1/2

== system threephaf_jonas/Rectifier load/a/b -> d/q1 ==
  vect : Inport  Port=1  LatchInput=off
  angle : Inport  Port=2  LatchInput=off
  Fcn_x : Fcn  Expr=u[1]*cos(u[3])-u[2]*sin(u[3])
  Fcn_y : Fcn  Expr=u[1]*sin(u[3])+u[2]*cos(u[3])
  Mux : Mux  Inputs=2
  Mux1 : Mux  Inputs=2
  Out : Outport  InitialOutput=0
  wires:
  Mux1/1 -> Out/1
  Fcn_y/1 -> Mux1/2
  Fcn_x/1 -> Mux1/1
  Mux/1 -> Fcn_y/1, Fcn_x/1
  angle/1 -> Mux/2
  vect/1 -> Mux/1

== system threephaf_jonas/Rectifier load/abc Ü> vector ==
  a : Inport  Port=1  LatchInput=off
  b : Inport  Port=2  LatchInput=off
  c : Inport  Port=3  LatchInput=off
  Fcn : Fcn  Expr=sqrt(3/2)*u[1]
  Fcn1 : Fcn  Expr=sqrt(1/2)*(u[1]-u[2])
  Gain : Gain  Gain=1/3
  Mux5 : Mux  Inputs=2
  Mux7 : Mux  Inputs=2
  Sum2 : Sum  Inputs=+++
  Ü> ua : Sum  Inputs=+-
  Ü> ub : Sum  Inputs=+-
  Ü> uc : Sum  Inputs=+-
  vect : Outport  InitialOutput=0
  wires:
  Fcn1/1 -> Mux5/2
  Fcn/1 -> Mux5/1
  Mux5/1 -> vect/1
  Mux7/1 -> Fcn1/1
  Ü> uc/1 -> Mux7/2
  Ü> ub/1 -> Mux7/1
  Ü> ua/1 -> Fcn/1
  Gain/1 -> Ü> uc/2, Ü> ub/2, Ü> ua/2
  a/1 -> Ü> ua/1, Sum2/1
  b/1 -> Ü> ub/1, Sum2/2
  Sum2/1 -> Gain/1
  c/1 -> Ü> uc/1, Sum2/3

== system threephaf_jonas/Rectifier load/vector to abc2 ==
  vect : Inport  Port=1  LatchInput=off
  Ü> a : Fcn  Expr=sqrt(2/3)*u[1]
  Ü> b : Fcn  Expr=-sqrt(1/6)*u[1]+sqrt(1/2)*u[2]
  Ü> c : Fcn  Expr=-sqrt(1/6)*u[1]-sqrt(1/2)*u[2]
  a : Outport  InitialOutput=0
  b : Outport  Port=2  InitialOutput=0
  c : Outport  Port=3  InitialOutput=0
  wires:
  vect/1 -> Ü> b/1, Ü> a/1, Ü> c/1
  Ü> b/1 -> b/1
  Ü> c/1 -> c/1
  Ü> a/1 -> a/1

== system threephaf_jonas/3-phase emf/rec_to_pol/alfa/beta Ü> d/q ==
  vect : Inport  Port=1  LatchInput=off
  angle : Inport  Port=2  LatchInput=off
  Fcn : Fcn  Expr=u[1]*cos(u[3])-u[2]*sin(u[3])
  Fcn1 : Fcn  Expr=u[1]*sin(u[3])+u[2]*cos(u[3])
  Mux : Mux  Inputs=2
  Mux1 : Mux  Inputs=2
  Out : Outport  InitialOutput=0
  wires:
  vect/1 -> Mux/1
  angle/1 -> Mux/2
  Mux/1 -> Fcn/1, Fcn1/1
  Fcn/1 -> Mux1/1
  Fcn1/1 -> Mux1/2
  Mux1/1 -> Out/1

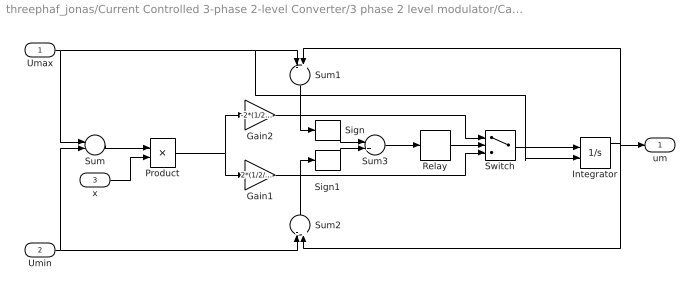
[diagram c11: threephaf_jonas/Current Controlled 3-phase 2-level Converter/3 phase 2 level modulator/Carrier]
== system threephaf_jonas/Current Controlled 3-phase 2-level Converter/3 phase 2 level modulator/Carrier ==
  Umax : Inport  Port=1  LatchInput=off
  Umin : Inport  Port=2  LatchInput=off
  x : Inport  Port=3  LatchInput=off
  Gain1 : Gain  Gain=2*(1/2/Ts)
  Gain2 : Gain  Gain=-2*(1/2/Ts)
  Integrator : Integrator  InitialConditionSource=external
  Product : Product
  Relay : Relay  OnSwitchValue=1  OffSwitchValue=-1  OffOutputValue=-1
  Sign : Signum
  Sign1 : Signum
  Sum : Sum  Inputs=+-
  Sum1 : Sum  Orientation=down  Inputs=-+
  Sum2 : Sum  Orientation=up  Inputs=-+
  Sum3 : Sum
  Switch : Switch
  um : Outport
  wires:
  Switch/1 -> Integrator/1
  Umax/1 -> Sum/1, Sum1/1, Integrator/2
  Umin/1 -> Sum/2, Sum2/1
  Gain2/1 -> Switch/1
  Gain1/1 -> Switch/3
  Integrator/1 -> Sum1/2, um/1, Sum2/2
  Sum1/1 -> Sign/1
  Sum2/1 -> Sign1/1
  Sign/1 -> Sum3/1
  Sign1/1 -> Sum3/2
  Sum3/1 -> Relay/1
  Relay/1 -> Switch/2
  Sum/1 -> Product/1
  Product/1 -> Gain2/1, Gain1/1
  x/1 -> Product/2

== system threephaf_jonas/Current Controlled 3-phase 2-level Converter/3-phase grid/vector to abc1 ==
  vect : Inport  Port=1  LatchInput=off
  Ü> a : Fcn  Expr=sqrt(2/3)*u[1]
  Ü> b : Fcn  Expr=-sqrt(1/6)*u[1]+sqrt(1/2)*u[2]
  Ü> c : Fcn  Expr=-sqrt(1/6)*u[1]-sqrt(1/2)*u[2]
  a : Outport  InitialOutput=0
  b : Outport  Port=2  InitialOutput=0
  c : Outport  Port=3  InitialOutput=0
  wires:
  vect/1 -> Ü> b/1, Ü> a/1, Ü> c/1
  Ü> b/1 -> b/1
  Ü> c/1 -> c/1
  Ü> a/1 -> a/1

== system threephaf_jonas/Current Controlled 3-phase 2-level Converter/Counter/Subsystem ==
  Trigger : TriggerPort  TriggerType=either
  Constant : Constant
  Memory : Memory  Orientation=left  InheritSampleTime=on
  Sum : Sum
  Out1 : Outport
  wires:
  Sum/1 -> Memory/1, Out1/1
  Memory/1 -> Sum/2
  Constant/1 -> Sum/1

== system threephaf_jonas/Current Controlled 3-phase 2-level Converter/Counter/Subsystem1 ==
  Trigger : TriggerPort  TriggerType=either
  Constant : Constant
  Memory : Memory  Orientation=left  InheritSampleTime=on
  Sum : Sum
  Out1 : Outport
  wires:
  Constant/1 -> Sum/1
  Memory/1 -> Sum/2
  Sum/1 -> Memory/1, Out1/1

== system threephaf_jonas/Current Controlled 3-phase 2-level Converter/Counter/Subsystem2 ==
  Trigger : TriggerPort  TriggerType=either
  Constant : Constant
  Memory : Memory  Orientation=left  InheritSampleTime=on
  Sum : Sum
  Out1 : Outport
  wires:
  Sum/1 -> Memory/1, Out1/1
  Memory/1 -> Sum/2
  Constant/1 -> Sum/1

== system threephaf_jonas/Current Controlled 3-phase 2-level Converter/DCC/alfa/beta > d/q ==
  vect : Inport  Port=1  LatchInput=off
  angle : Inport  Port=2  LatchInput=off
  Fcn : Fcn  Expr=u[1]*cos(u[3])-u[2]*sin(u[3])
  Fcn1 : Fcn  Expr=u[1]*sin(u[3])+u[2]*cos(u[3])
  Mux : Mux  Inputs=2
  Mux1 : Mux  Inputs=2
  Out : Outport  InitialOutput=0
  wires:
  vect/1 -> Mux/1
  angle/1 -> Mux/2
  Mux/1 -> Fcn/1, Fcn1/1
  Fcn/1 -> Mux1/1
  Fcn1/1 -> Mux1/2
  Mux1/1 -> Out/1

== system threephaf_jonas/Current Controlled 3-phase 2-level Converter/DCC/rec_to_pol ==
  rect : Inport  Port=1  LatchInput=off
  Derivative : Derivative
  Gain : Gain  Gain=-1
  alfa/beta Ü> d/q : Subsystem
  "angle " : Fcn  Expr=atan2(u[2],u[1])
  "mod " : Fcn  Expr=sqrt(u[1]^2+u[2]^2)
  mod : Outport  InitialOutput=0
  angle : Outport  Port=2  InitialOutput=0
  emf : Outport  Port=3  InitialOutput=0
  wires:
  "angle "/1 -> angle/1, Gain/1
  rect/1 -> "angle "/1, "mod "/1, Derivative/1
  "mod "/1 -> mod/1
  Gain/1 -> alfa/beta Ü> d/q/2(angle)
  Derivative/1 -> alfa/beta Ü> d/q/1(vect)
  alfa/beta Ü> d/q/1(Out) -> emf/1

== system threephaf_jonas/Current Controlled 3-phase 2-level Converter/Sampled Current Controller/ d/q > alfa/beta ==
  vect : Inport  Port=1  LatchInput=off
  angle : Inport  Port=2  LatchInput=off
  Fcn : Fcn  Expr=u[1]*cos(u[3])-u[2]*sin(u[3])
  Fcn1 : Fcn  Expr=u[1]*sin(u[3])+u[2]*cos(u[3])
  Mux : Mux  Inputs=2
  Mux1 : Mux  Inputs=2
  Out : Outport  InitialOutput=0
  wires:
  Mux1/1 -> Out/1
  Fcn1/1 -> Mux1/2
  Fcn/1 -> Mux1/1
  Mux/1 -> Fcn1/1, Fcn/1
  angle/1 -> Mux/2
  vect/1 -> Mux/1

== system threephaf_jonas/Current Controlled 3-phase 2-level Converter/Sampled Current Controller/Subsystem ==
  u : Inport  Orientation=left  Port=1  LatchInput=off
  Gammalt mätvärde2 : UnitDelay  Orientation=down  SampleTime=Ts
  Gammalt mätvärde3 : UnitDelay  Orientation=left  SampleTime=Ts
  Matsprediktor1 : Sum  Orientation=left  Inputs=+-
  Proportional3 : Gain  Orientation=left  Gain=Ts/L
  Proportional4 : Gain  Orientation=left  Gain=(1-Ts/(L/R))
  Sum1 : Sum  Orientation=left
  di_smith : Outport  Orientation=left
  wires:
  Proportional3/1 -> Sum1/1
  Proportional4/1 -> Sum1/2
  Sum1/1 -> Gammalt mätvärde2/1, Matsprediktor1/1
  u/1 -> Proportional3/1
  Matsprediktor1/1 -> Gammalt mätvärde3/1
  Gammalt mätvärde3/1 -> di_smith/1
  Gammalt mätvärde2/1 -> Proportional4/1, Matsprediktor1/2

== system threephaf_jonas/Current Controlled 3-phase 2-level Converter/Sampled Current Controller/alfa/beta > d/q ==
  vect : Inport  Port=1  LatchInput=off
  angle : Inport  Port=2  LatchInput=off
  Fcn : Fcn  Expr=u[1]*cos(u[3])-u[2]*sin(u[3])
  Fcn1 : Fcn  Expr=u[1]*sin(u[3])+u[2]*cos(u[3])
  Mux : Mux  Inputs=2
  Mux1 : Mux  Inputs=2
  Out : Outport  InitialOutput=0
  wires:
  vect/1 -> Mux/1
  angle/1 -> Mux/2
  Mux/1 -> Fcn/1, Fcn1/1
  Fcn/1 -> Mux1/1
  Fcn1/1 -> Mux1/2
  Mux1/1 -> Out/1

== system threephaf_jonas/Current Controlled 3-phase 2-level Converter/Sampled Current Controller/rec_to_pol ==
  rect : Inport  Port=1  LatchInput=off
  Derivative : Derivative
  Gain : Gain  Gain=-1
  alfa/beta Ü> d/q : Subsystem
  "angle " : Fcn  Expr=atan2(u[2],u[1])
  "mod " : Fcn  Expr=sqrt(u[1]^2+u[2]^2)
  e : Outport  InitialOutput=0
  angle : Outport  Port=2  InitialOutput=0
  mod : Outport  Port=3  InitialOutput=0
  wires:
  "angle "/1 -> angle/1, Gain/1
  rect/1 -> "angle "/1, "mod "/1, Derivative/1
  "mod "/1 -> mod/1
  Gain/1 -> alfa/beta Ü> d/q/2(angle)
  Derivative/1 -> alfa/beta Ü> d/q/1(vect)
  alfa/beta Ü> d/q/1(Out) -> e/1

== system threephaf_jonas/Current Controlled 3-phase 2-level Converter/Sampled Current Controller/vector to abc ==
  vect : Inport  Port=1  LatchInput=off
  Ü> a : Fcn  Expr=sqrt(2/3)*u[1]
  Ü> b : Fcn  Expr=-sqrt(1/6)*u[1]+sqrt(1/2)*u[2]
  Ü> c : Fcn  Expr=-sqrt(1/6)*u[1]-sqrt(1/2)*u[2]
  a : Outport  InitialOutput=0
  b : Outport  Port=2  InitialOutput=0
  c : Outport  Port=3  InitialOutput=0
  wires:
  vect/1 -> Ü> b/1, Ü> a/1, Ü> c/1
  Ü> b/1 -> b/1
  Ü> c/1 -> c/1
  Ü> a/1 -> a/1

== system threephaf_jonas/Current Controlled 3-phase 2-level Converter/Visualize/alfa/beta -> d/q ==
  vect : Inport  Port=1  LatchInput=off
  angle : Inport  Port=2  LatchInput=off
  Fcn : Fcn  Expr=u[1]*cos(u[3])-u[2]*sin(u[3])
  Fcn1 : Fcn  Expr=u[1]*sin(u[3])+u[2]*cos(u[3])
  Mux : Mux  Inputs=2
  Mux1 : Mux  Inputs=2
  Out : Outport  InitialOutput=0
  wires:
  vect/1 -> Mux/1
  angle/1 -> Mux/2
  Mux/1 -> Fcn/1, Fcn1/1
  Fcn/1 -> Mux1/1
  Fcn1/1 -> Mux1/2
  Mux1/1 -> Out/1

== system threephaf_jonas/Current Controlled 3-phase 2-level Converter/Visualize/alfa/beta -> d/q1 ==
  vect : Inport  Port=1  LatchInput=off
  angle : Inport  Port=2  LatchInput=off
  Fcn : Fcn  Expr=u[1]*cos(u[3])-u[2]*sin(u[3])
  Fcn1 : Fcn  Expr=u[1]*sin(u[3])+u[2]*cos(u[3])
  Mux : Mux  Inputs=2
  Mux1 : Mux  Inputs=2
  Out : Outport  InitialOutput=0
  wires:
  Mux1/1 -> Out/1
  Fcn1/1 -> Mux1/2
  Fcn/1 -> Mux1/1
  Mux/1 -> Fcn1/1, Fcn/1
  angle/1 -> Mux/2
  vect/1 -> Mux/1

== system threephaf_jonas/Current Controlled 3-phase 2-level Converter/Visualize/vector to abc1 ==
  vect : Inport  Port=1  LatchInput=off
  Ü> a : Fcn  Expr=sqrt(2/3)*u[1]
  Ü> b : Fcn  Expr=-sqrt(1/6)*u[1]+sqrt(1/2)*u[2]
  Ü> c : Fcn  Expr=-sqrt(1/6)*u[1]-sqrt(1/2)*u[2]
  a : Outport  InitialOutput=0
  b : Outport  Port=2  InitialOutput=0
  c : Outport  Port=3  InitialOutput=0
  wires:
  Ü> a/1 -> a/1
  Ü> c/1 -> c/1
  Ü> b/1 -> b/1
  vect/1 -> Ü> c/1, Ü> a/1, Ü> b/1

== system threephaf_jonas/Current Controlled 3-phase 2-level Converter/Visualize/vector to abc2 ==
  vect : Inport  Port=1  LatchInput=off
  Ü> a : Fcn  Expr=sqrt(2/3)*u[1]
  Ü> b : Fcn  Expr=-sqrt(1/6)*u[1]+sqrt(1/2)*u[2]
  Ü> c : Fcn  Expr=-sqrt(1/6)*u[1]-sqrt(1/2)*u[2]
  a : Outport  InitialOutput=0
  b : Outport  Port=2  InitialOutput=0
  c : Outport  Port=3  InitialOutput=0
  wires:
  vect/1 -> Ü> b/1, Ü> a/1, Ü> c/1
  Ü> b/1 -> b/1
  Ü> c/1 -> c/1
  Ü> a/1 -> a/1
